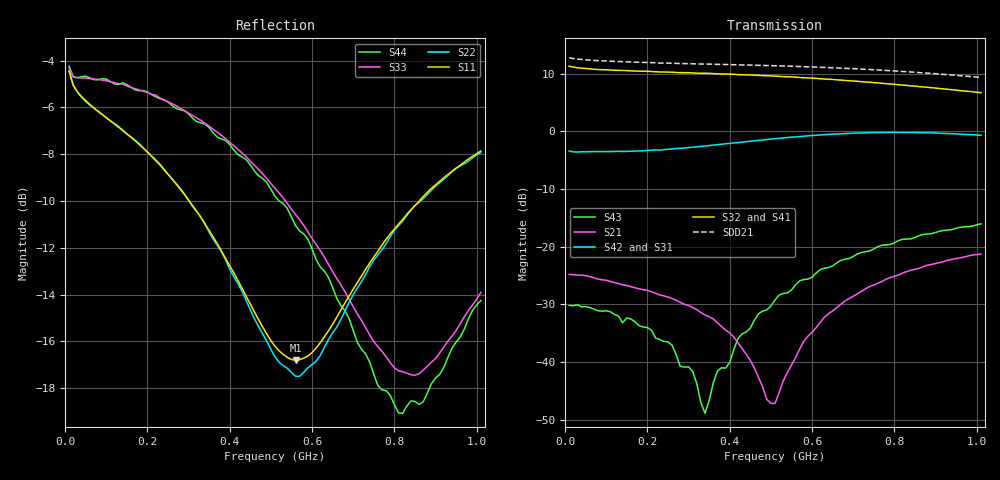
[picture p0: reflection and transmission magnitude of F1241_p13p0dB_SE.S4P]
! Integrated Device Technology
! Corporate Headquarters
! 6024 Silver Creek Valley Road
! San Jose, CA 95138  USA
! Phone:  1-408-284-8200
! Toll Free:  1-800-223-1366
! Webpage:  http://www.idt.com/
! Timing and RF Division
! 515 Groton Road, Suite 102
! Westford, MA 01886-6024
! Device:  F1241
! Description: Dual Intermediate Frequency Digital Variable Gain Amplifier
! Frequency:  10.0 -  500.00 MHz
! Package:  5x5 mm QFN Plastic Package: 32 pin
! Ports:  8 RF, 20 DC
!  Pin  1  = GA3  Pin 17  = RF OUT_B+
!  Pin  2  = GA4  Pin 18  = RF OUT_B-
!  Pin  3  = GA5  Pin 19  = STBY_B
!  Pin  4  = ISET_A  Pin 20  = Ground
!  Pin  5  = ISET_B  Pin 21  = Ground
!  Pin  6  = GB5  Pin 22  = STB_A
!  Pin  7  = GB4  Pin 23  = RF OUT_A-  = Port 4
!  Pin  8  = GB3  Pin 24  = RF OUT_A+  = Port 3
!  Pin  9  = GB2  Pin 25  = NO CONNECT
!  Pin 10  = GB1  Pin 26  = NO CONNECT
!  Pin 11  = RF IN_B+  Pin 27  = VCC
!  Pin 12  = RF IN_B-  Pin 28  = Ground
!  Pin 13  = Ground  Pin 29  = RF IN_A-  = Port 2
!  Pin 14  = VCC  Pin 30  = RF IN_A+  = Port 1
!  Pin 15  = NO CONNECT  Pin 31  = GA1
!  Pin 16  = NO CONNECT  Pin 32  = GA2
! State:  7
! Gain State:  13.0 dB
! Voltages:  Vcc = +5.00 Volts  Icc approximately 160.0 mA or 80 mA per channel.
! Data:  The device was measured on a custom evaluation board which has
!  individual transmission lines to the RF pins.  Data was collected
!  using a calibrated network analyzer.  The evaluation board was
!  de-embedded using a port reference technique.
!  The reference plane is the edge of the package pin.
!  Only Channel A was measured.
!  This data is in single-ended operation.  If your needs are balanced
!  or differential S-parameters then this file needs to be used a
!  linear simulator.
! Misc:  Lot Code  160028MY
!  Action Tracker AT004
! Date Measured:  2014-08-14
! Date:  2014-08-28  MJV
! Note:
!  Integrated Device Technology supplies this data as a sample of measured
!  data at the package pin for this product.  Your particular data for this
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# Hz S dB R 50
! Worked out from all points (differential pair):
!   101 points, 10 MHz to 1.01 GHz, reference 50 ohm
!   strongest paths, dB at 10 MHz, 260 MHz, 510 MHz, 760 MHz, 1.01 GHz:
!     S32: 11.3, 10.3, 9.6, 8.4, 6.7
!     S41: 11.3, 10.2, 9.5, 8.2, 6.5
!     S42: -3.4, -3.0, -1.3, -0.2, -0.7
!     S31: -3.4, -3.1, -1.5, -0.4, -0.8
!     S21: -24.8, -29.0, -47.2, -26.3, -21.3
!     S43: -30.2, -37.1, -29.2, -20.0, -16.0
!   taken as a pair (ports 2,1 in; 3,4 out), SDD21 dB: 12.8, 11.8, 11.4, 10.7, 9.3
!   lowest |S11| = -16.8 dB at 560 MHz (marker M1), VSWR 1.34, Z = 39.6 - j7.72 ohm
!   |S11| at or under -10 dB: 301.8 MHz to 860.2 MHz (558.4 MHz wide, 96.1 % of centre)
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1e7  -4.45 -14.5  -24.85 6.9  -48.99 41.9  -20.58 9.5
     -24.81 6.7  -4.46 -14.3  -20.59 9.2  -48.88 42.0
     -3.42 1.8  11.31 -177.1  -4.31 -11.7  -30.26 24.3
     11.34 -177.0  -3.41 1.9  -30.19 23.3  -4.24 -11.8
3.4e8  -10.98 -59.8  -31.43 -43.3  -29.77 46.0  -20.74 -14.5
       -31.83 -49.3  -10.98 -57.2  -20.67 -14.5  -29.75 45.0
       -2.72 -17.2  10.07 133.6  -6.67 -30.6  -38.20 -107.6
       10.00 132.7  -2.53 -17.7  -48.90 -115.4  -6.71 -29.1
4.3e8  -13.73 -82.1  -36.97 -52.8  -28.00 37.1  -20.41 -19.6
       -37.65 -70.8  -13.85 -78.8  -20.31 -19.4  -27.95 36.1
       -2.08 -23.5  9.83 122.0  -7.94 -39.5  -35.07 -170.1
       9.74 121.1  -1.86 -24.6  -35.11 150.7  -8.11 -37.5
4.9e8  -15.68 -104.2  -46.42 -59.5  -27.06 31.4  -20.22 -23.3
       -46.47 -120.7  -15.99 -101.0  -20.08 -23.3  -27.01 29.8
       -1.64 -28.8  9.65 114.2  -9.04 -46.3  -30.84 162.4
       9.55 113.3  -1.41 -30.2  -30.97 136.1  -9.20 -44.3
5.1e8  -16.21 -113.3  -63.13 -78.2  -26.81 29.3  -20.14 -24.8
       -47.19 -162.0  -16.66 -110.3  -20.00 -24.6  -26.74 27.9
       -1.49 -30.7  9.59 111.6  -9.46 -48.7  -30.15 155.4
       9.47 110.7  -1.27 -32.3  -29.23 136.3  -9.80 -46.6
5.6e8  -16.80 -138.6  -41.72 110.4  -26.21 24.3  -20.04 -28.4
       -39.22 136.6  -17.49 -137.1  -19.85 -28.3  -26.15 22.6
       -1.16 -35.9  9.41 105.1  -10.58 -55.5  -27.58 142.8
       9.27 104.3  -0.94 -37.7  -26.59 127.1  -11.06 -52.9
1.01e9  -7.86 122.1  -21.92 62.0  -23.77 -15.1  -20.76 -63.1
        -21.26 62.7  -7.93 121.9  -20.22 -63.5  -23.66 -19.1
        -0.85 -92.4  6.71 51.0  -13.91 173.3  -16.68 68.7
        6.49 50.3  -0.67 -95.7  -16.03 60.7  -14.25 165.7
